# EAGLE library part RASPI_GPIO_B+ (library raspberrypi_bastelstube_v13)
Only the 2x20 header connector, nothing else
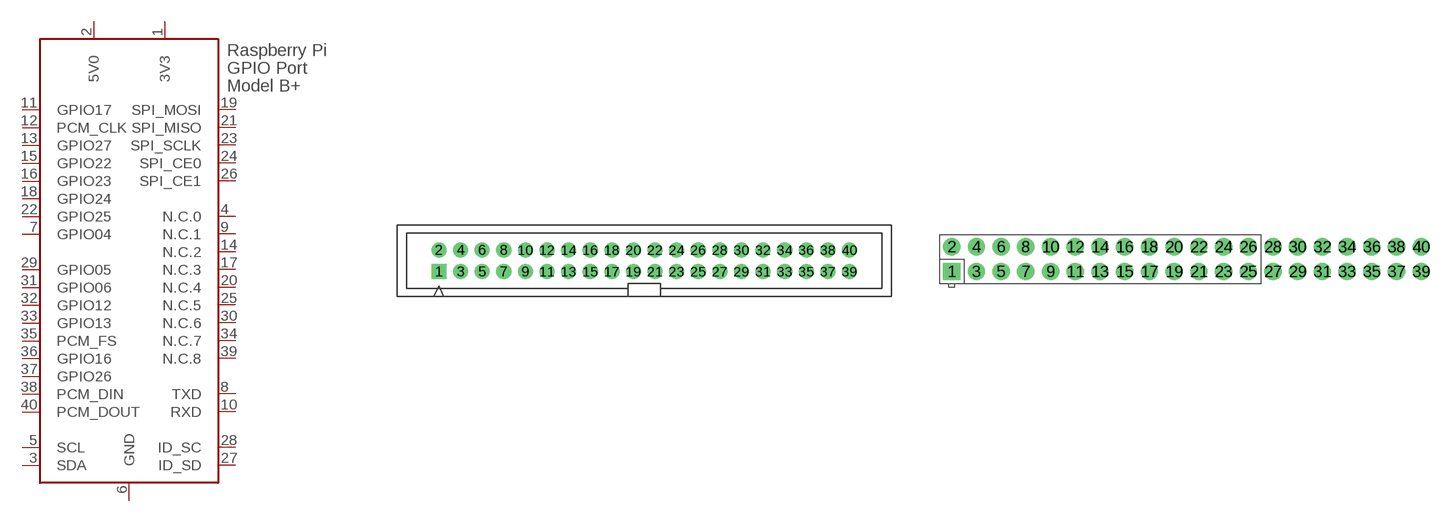
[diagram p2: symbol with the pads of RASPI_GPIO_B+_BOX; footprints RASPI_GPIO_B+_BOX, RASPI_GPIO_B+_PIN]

Designator prefix X

## RASPI_GPIO_B+_BOX  [RASPI_GPIO_B+_BOX]
1  3V3  pwr
2  5V0  pwr
3  SDA
4  N.C.0  nc
5  SCL
6  GND  pwr
7  GPIO04
8  TXD
9  N.C.1  nc
10  RXD
11  GPIO17
12  PCM_CLK
13  GPIO27
14  N.C.2  nc
15  GPIO22
16  GPIO23
17  N.C.3  nc
18  GPIO24
19  SPI_MOSI
20  N.C.4  nc
21  SPI_MISO
22  GPIO25
23  SPI_SCLK
24  SPI_CE0
25  N.C.5  nc
26  SPI_CE1
27  ID_SD  nc
28  ID_SC  nc
29  GPIO05  nc
30  N.C.6  nc
31  GPIO06  nc
32  GPIO12  nc
33  GPIO13  nc
34  N.C.7  nc
35  PCM_FS  nc
36  GPIO16  nc
37  GPIO26  nc
38  PCM_DIN  nc
39  N.C.8  nc
40  PCM_DOUT  nc

## RASPI_GPIO_B+_PIN  [RASPI_GPIO_B+_PIN]
Pads as for RASPI_GPIO_B+_BOX

## Footprint RASPI_GPIO_B+_BOX (pad centres in mm)
40-pin box header for Raspberry Pi GPIO model B+ for use with flat ribbon cables
drill 1 pad 1.778 square: 1 -24.13,-1.27
drill 1 pad 1.778: 2 -24.13,1.27; 3 -21.59,-1.27; 4 -21.59,1.27; 5 -19.05,-1.27; 6 -19.05,1.27; 7 -16.51,-1.27; 8 -16.51,1.27; 9 -13.97,-1.27; 10 -13.97,1.27; 11 -11.43,-1.27; 12 -11.43,1.27; 13 -8.89,-1.27; 14 -8.89,1.27; 15 -6.35,-1.27; 16 -6.35,1.27; 17 -3.81,-1.27; 18 -3.81,1.27; 19 -1.27,-1.27; 20 -1.27,1.27; 21 1.27,-1.27; 22 1.27,1.27; 23 3.81,-1.27; 24 3.81,1.27; 25 6.35,-1.27; 26 6.35,1.27; 27 8.89,-1.27; 28 8.89,1.27; 29 11.43,-1.27; 30 11.43,1.27; 31 13.97,-1.27; 32 13.97,1.27; 33 16.51,-1.27; 34 16.51,1.27; 35 19.05,-1.27; 36 19.05,1.27; 37 21.59,-1.27; 38 21.59,1.27; 39 24.13,-1.27; 40 24.13,1.27

## Footprint RASPI_GPIO_B+_PIN (pad centres in mm)
40-pin connector for Raspberry Pi GPIO model B+ just the two rows of pins
drill 1 pad 1.778 square: 1 -24.13,-1.27
drill 1 pad 1.778: 2 -24.13,1.27; 3 -21.59,-1.27; 4 -21.59,1.27; 5 -19.05,-1.27; 6 -19.05,1.27; 7 -16.51,-1.27; 8 -16.51,1.27; 9 -13.97,-1.27; 10 -13.97,1.27; 11 -11.43,-1.27; 12 -11.43,1.27; 13 -8.89,-1.27; 14 -8.89,1.27; 15 -6.35,-1.27; 16 -6.35,1.27; 17 -3.81,-1.27; 18 -3.81,1.27; 19 -1.27,-1.27; 20 -1.27,1.27; 21 1.27,-1.27; 22 1.27,1.27; 23 3.81,-1.27; 24 3.81,1.27; 25 6.35,-1.27; 26 6.35,1.27; 27 8.89,-1.27; 28 8.89,1.27; 29 11.43,-1.27; 30 11.43,1.27; 31 13.97,-1.27; 32 13.97,1.27; 33 16.51,-1.27; 34 16.51,1.27; 35 19.05,-1.27; 36 19.05,1.27; 37 21.59,-1.27; 38 21.59,1.27; 39 24.13,-1.27; 40 24.13,1.27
